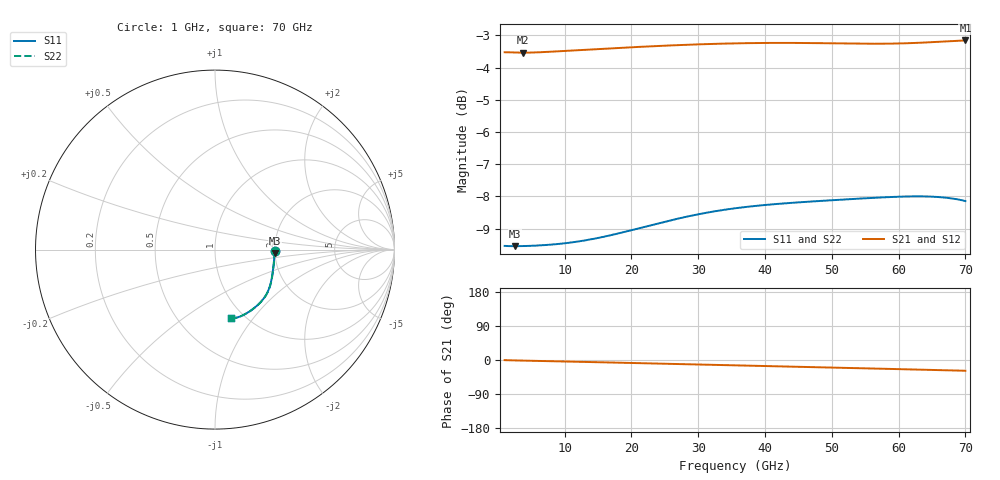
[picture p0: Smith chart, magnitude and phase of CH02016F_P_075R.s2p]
# GHz S RI R 75
! S-Parameters data
! Freq  reS11  imS11  reS21  imS21  reS12  imS12  reS22  imS22
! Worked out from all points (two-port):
!   401 points, 1 GHz to 70 GHz, reference 75 ohm
!   highest |S21| = -3.16 dB at 70 GHz (marker M1); lowest = -3.5 dB at 3.76 GHz (marker M2)
!   |S21| within 3 dB of the highest: start of sweep to end of sweep
!   lowest |S11| = -9.5 dB at 2.553 GHz (marker M3), VSWR 2.00, Z = 149 - j7.05 ohm
!   |S11| at or under -10 dB: nowhere
!   |S22| runs from -9.5 to -8.0 dB; largest |S21 - S12| = 0
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1  0.3333 -0.00792  0.6666 -0.00449  0.6666 -0.00449  0.3333 -0.00798
2.5525  0.3324 -0.021  0.6658 -0.0131  0.6658 -0.0131  0.3325 -0.0211
3.76  0.3318 -0.0304  0.6654 -0.0182  0.6654 -0.0182  0.3319 -0.0306
8.4175  0.3287 -0.0661  0.6673 -0.0373  0.6673 -0.0373  0.3289 -0.0665
12.5575  0.325 -0.0977  0.6698 -0.0565  0.6698 -0.0565  0.3255 -0.0982
17.0425  0.3205 -0.1322  0.6715 -0.0787  0.6715 -0.0787  0.3213 -0.1326
24.115  0.3108 -0.1849  0.6723 -0.114  0.6723 -0.114  0.3118 -0.1852
27.0475  0.3052 -0.2052  0.6718 -0.1282  0.6718 -0.1282  0.3062 -0.2054
29.98  0.2984 -0.2243  0.6708 -0.1422  0.6708 -0.1422  0.2994 -0.2243
32.74  0.2908 -0.2411  0.6694 -0.1551  0.6694 -0.1551  0.2917 -0.2411
35.5  0.2819 -0.257  0.6674 -0.1679  0.6674 -0.1679  0.2827 -0.2569
38.4325  0.2708 -0.2731  0.6646 -0.1815  0.6646 -0.1815  0.2714 -0.273
41.1925  0.2588 -0.2877  0.6613 -0.1944  0.6613 -0.1944  0.2593 -0.2876
43.9525  0.2453 -0.3018  0.6574 -0.2073  0.6574 -0.2073  0.2458 -0.3018
47.0575  0.2287 -0.317  0.6522 -0.2219  0.6522 -0.2219  0.2291 -0.3171
53.095  0.1934 -0.3436  0.6408 -0.2493  0.6408 -0.2493  0.1938 -0.3438
55.855  0.1766 -0.3542  0.6355 -0.2616  0.6355 -0.2616  0.1771 -0.3544
58.615  0.1597 -0.3635  0.6304 -0.2742  0.6304 -0.2742  0.1602 -0.3638
62.065  0.1381 -0.3733  0.6246 -0.2907  0.6246 -0.2907  0.1387 -0.3736
64.9975  0.1194 -0.3793  0.6199 -0.3056  0.6199 -0.3056  0.1201 -0.3796
67.585  0.103 -0.382  0.6158 -0.319  0.6158 -0.319  0.1037 -0.3822
70  0.0886 -0.3813  0.6118 -0.3304  0.6118 -0.3304  0.0893 -0.3815
